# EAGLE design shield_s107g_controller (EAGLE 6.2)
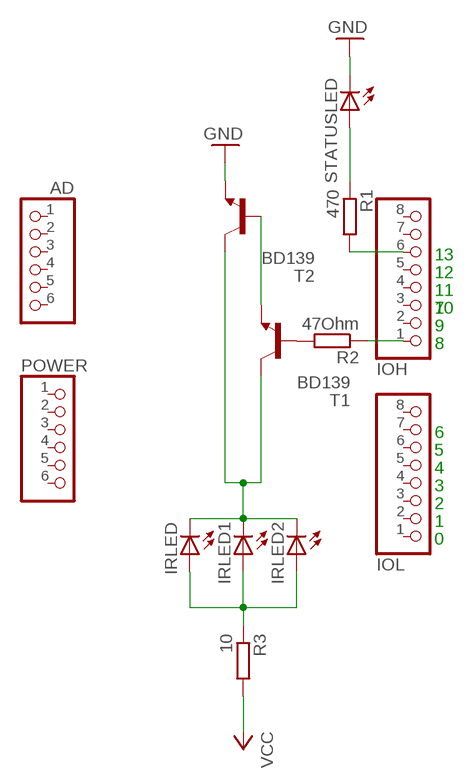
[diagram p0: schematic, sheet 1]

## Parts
AD  PINHD-1X6  [1X06]
IOH  PINHD-1X8  [1X08]
IOL  PINHD-1X8  [1X08]
IRLED  LED3MM  [LED3MM]
IRLED1  LED3MM  [LED3MM]
IRLED2  LED3MM  [LED3MM]
POWER  PINHD-1X6  [1X06]
R1  470  R-EU_0207/7  [0207/7]
R2  47Ohm  R-EU_0207/7  [0207/7]
R3  10  R-EU_0207/7  [0207/7]
STATUSLED  LED3MM  [LED3MM]
T1  BD139  [TO126]
T2  BD139  [TO126]

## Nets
GND: STATUSLED.K(C) T2.1(E)
N$1: IOH.1 R2.1
N$2: R2.2 T1.3(B)
N$3: T1.1(E) T2.3(B)
N$4: R1.1 STATUSLED.A
N$5: IRLED1.A IRLED2.A IRLED.A R3.1
N$6: IOH.6 R1.2
N$7: IRLED1.K(C) IRLED2.K(C) IRLED.K(C) T1.2(C) T2.2(C)
VCC: R3.2
Unconnected: AD.1 AD.2 AD.3 AD.4 AD.5 AD.6 IOH.2 IOH.3 IOH.4 IOH.5 IOH.7 IOH.8 IOL.1 IOL.2 IOL.3 IOL.4 IOL.5 IOL.6 IOL.7 IOL.8 POWER.1 POWER.2 POWER.3 POWER.4 POWER.5 POWER.6

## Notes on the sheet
- 13
- 12
- 11
- 10 | 7
- 9
- 8
- 6
- 5
- 4
- 3
- 2
- 1
- 0

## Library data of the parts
AD POWER = pinhead:PINHD-1X6: PIN HEADER
IOH IOL = pinhead:PINHD-1X8: PIN HEADER
IRLED IRLED1 IRLED2 STATUSLED = led:LED: LED
R1-R3 = rcl:R-EU_: RESISTOR, European symbol
T1 T2 = transistor:BD139: NPN TRANSISTOR

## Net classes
0 default: width 0.152 mm, drill 0.305 mm, clearance 0.152 mm

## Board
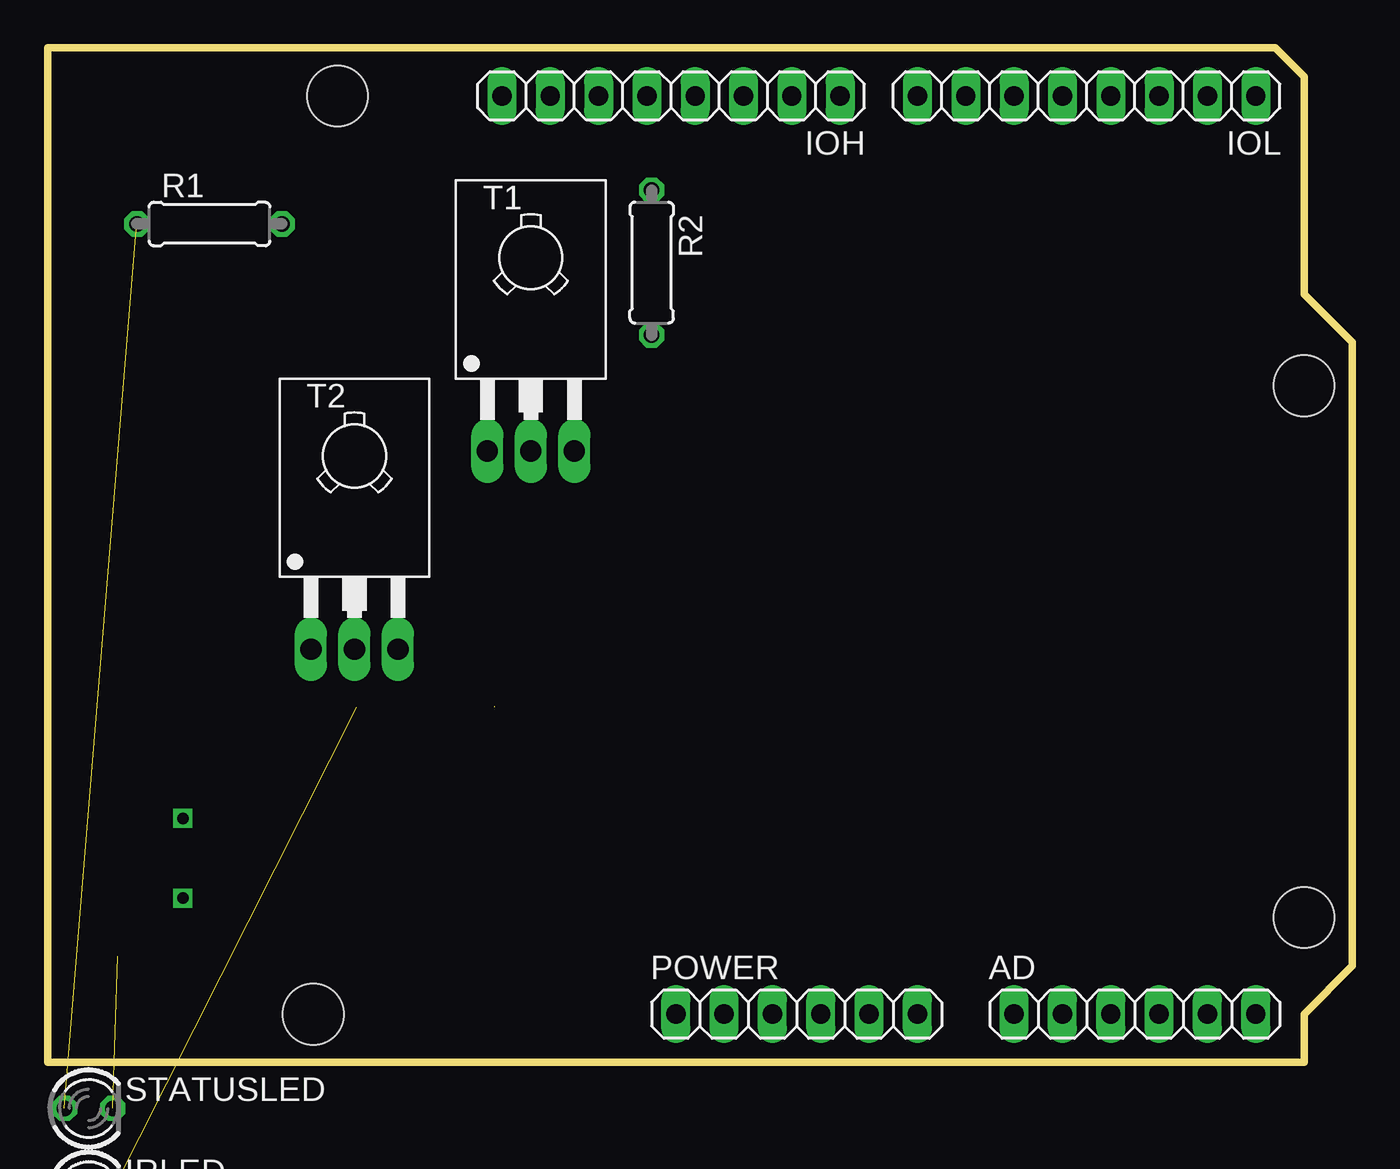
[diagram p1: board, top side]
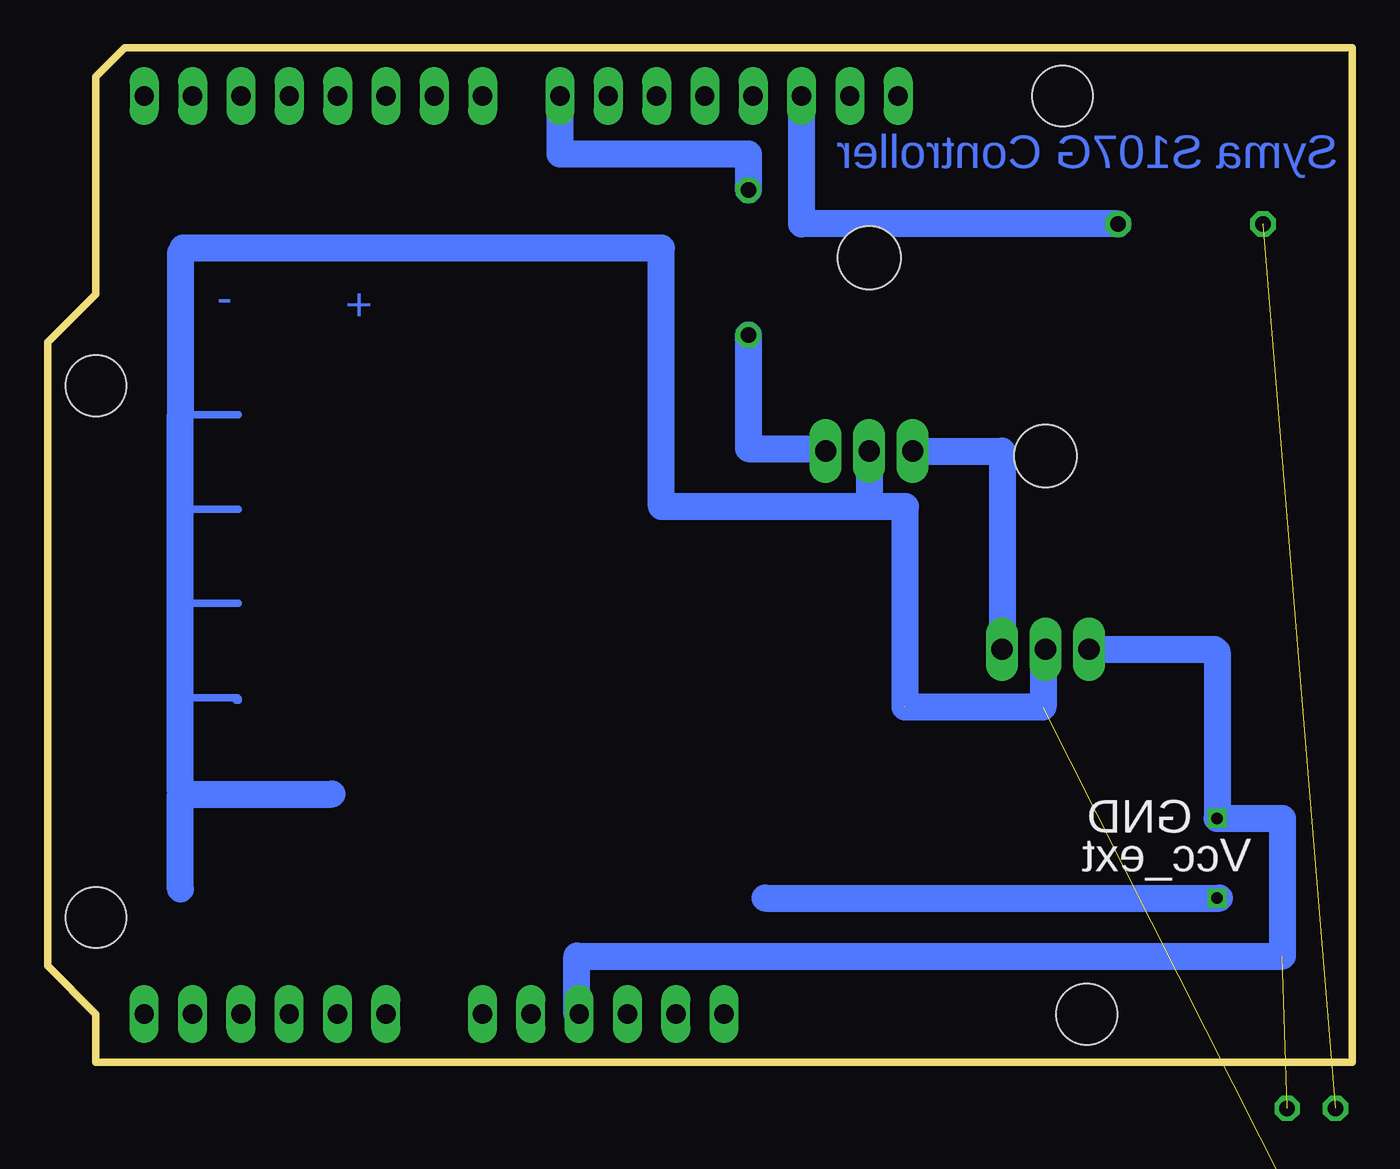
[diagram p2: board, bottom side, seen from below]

Size 68.58 x 53.34 mm. Coordinates in mm from the lower left corner, seen from the top.
Outline: 0,0 0,53.34 64.52,53.34 66.04,51.82 66.04,40.39 68.58,37.85 68.58,5.08 66.04,2.54 66.04,0 0,0
Copper layers (1*16): Top 0.035mm / dielectric 1.5mm / Bottom 0.035mm
Design rules: minimum track width 16mil, minimum drill 24mil, track to track 8mil, track to pad 8mil, pad to pad 8mil, via to via 8mil, smd to smd 8mil, copper to edge 30mil, drill to drill 8mil, minimum pad ring 10mil, minimum via ring 8mil, stop-mask expansion 2mil, vias tented up to drill 0mil, thermal gap 10mil
Holes 3.2 mm at 66.04,35.56 66.04,7.62 15.24,50.8 13.97,2.54

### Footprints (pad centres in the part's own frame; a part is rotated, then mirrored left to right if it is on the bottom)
1X06 = drill 1.016 long: 1 -6.35,0; 2 -3.81,0; 3 -1.27,0; 4 1.27,0; 5 3.81,0; 6 6.35,0
1X08 = drill 1.016 long: 1 -8.89,0; 2 -6.35,0; 3 -3.81,0; 4 -1.27,0; 5 1.27,0; 6 3.81,0; 7 6.35,0; 8 8.89,0
LED3MM = drill 0.813 octagon: A -1.27,0; K 1.27,0
0207/7 = drill 0.813 octagon: 1 -3.81,0; 2 3.81,0
TO126 = drill 1.118 long: 1 -2.286,-5.08; 2 0,-5.08; 3 2.286,-5.08 | hole 3.302: 0,5.08

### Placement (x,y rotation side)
AD  57.15,2.54 0 top
IOH  32.77,50.8 180 top
IOL  54.61,50.8 180 top
IRLED  not placed on the board
IRLED1  not placed on the board
IRLED2  not placed on the board
POWER  39.37,2.54 0 top
R1  8.51,44.07 0 top
R2  31.75,42.04 270 top
R3  not placed on the board
STATUSLED  2.16,-2.41 0 top
T1  25.4,37.21 0 top
T2  16.13,26.8 0 top

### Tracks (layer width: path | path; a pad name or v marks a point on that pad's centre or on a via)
GND  (1 unrouted)
  Bottom 0.406: 7.09,21.82 6.99,21.72 T2.1 | 7.24,21.72 7.11,21.59 | 5.21,12.57 3.68,12.83
  Bottom 1.422: T2.1 7.24,21.72 | 7.11,21.59 7.11,12.83 3.68,12.83 3.68,5.59 40.77,5.59 40.77,2.54
N$1
  Bottom 0.406: 31.88,47.75 31.75,47.75
  Bottom 1.422: IOH.1 41.66,47.75 31.88,47.75 | 31.75,47.75 R2.1
N$2
  Bottom 0.406: 27.69,32.26 T1.3
  Bottom 1.422: R2.2 31.75,32.26 27.69,32.26
N$3
  Bottom 1.422: T1.1 18.41,32.13 T2.3
N$4  (1 unrouted)
N$5  (3 unrouted)
N$6
  Bottom 1.422: IOH.6 28.96,44.07 R1.2
N$7  (4 unrouted)
  Bottom 0.406: 61.59,14.1 61.59,19.11 61.59,24.26 | 61.34,24.11 61.34,24.26 61.59,24.26 | 61.59,29.11 61.72,29.21 61.59,29.21 | 61.59,29.21 61.59,29.11 | 61.59,29.11 61.59,24.26 | 61.59,34.11 61.59,29.21 | 61.47,42.8 61.47,42.55 61.59,42.55 | T2.2 16.26,21.72
  Bottom 1.422: 23.5,18.71 23.5,29.21 25.4,29.21 | T1.2 25.4,29.21 | 25.4,29.21 36.32,29.21 36.32,42.8 61.47,42.8 | 61.59,9.11 61.59,14.1 53.63,14.1 | 61.59,42.55 61.59,34.11 | 16.26,21.72 16.26,18.67 23.52,18.67
N$9  (via drill 0.6)
  other vias: 7.11,8.64
N$13  (via drill 0.6)
  other vias: 7.11,12.83
N$21
  Bottom 1.422: 30.86,8.64 6.99,8.64
N$22
  Bottom 0.406: 61.59,11.81 61.59,13.97 | 61.59,13.97 61.59,14.1 61.47,14.1 | 58.55,14.1 61.47,14.1 | 61.47,14.1 arc-90 61.59,13.97
N$23
  Bottom 0.406: 61.59,19.18 58.8,19.18 | 58.8,19.18 58.67,19.18 arc90 58.55,19.05 58.67,19.05 arc-90 58.8,19.18 | 61.59,24.13 58.55,24.13 | 61.59,29.08 58.55,29.08 | 61.59,34.04 58.55,34.04
  Bottom 1.422: 61.59,14.22 61.59,19.18 61.59,24.13 61.59,29.08 61.59,34.04

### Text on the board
Bottom: Syma S107G Controller | + | -
bNames: GND | Vcc_ext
